{attribute 'no_assign'}
FUNCTION_BLOCK FB_LN_IED_MUnn_LLN0 EXTENDS FB_AcsiCommonLogicalNodeClass
VAR_INPUT
	NamPlt: FB_DO_IED_MUnn_LLN0_NamPlt := (sClass:='LPL', bLinkResult:=THIS^.AddDataToContainer(ipData:=NamPlt));
	Beh: FB_DO_IED_MUnn_LLN0_Beh := (sClass:='ENS', bLinkResult:=THIS^.AddDataToContainer(ipData:=Beh));
	Health: FB_DO_IED_MUnn_LLN0_Health := (sClass:='ENS', bLinkResult:=THIS^.AddDataToContainer(ipData:=Health));
	Mod_: FB_DO_IED_MUnn_LLN0_Mod := (sObjectName:='Mod', sClass:='ENC', bLinkResult:=THIS^.AddDataToContainer(ipData:=Mod_));
	
	PhsMeas1: FB_DS_IED_MUnn_LLN0_PhsMeas1 := (bLinkResult:=THIS^.AddDataSetToContainer(ipDataSet:=PhsMeas1));
	
	MSVCB01: FB_GseMsvCBImplClass := (MsvID:=(sValue:='xxxxMUnn01'), DatSet:=(sValue:='IEDMUnn/LLN0.PhsMeas1'), ConfRev:=(nValue:=1), SmpRate:=(nValue:=80), OptFlds:=(RefreshTime:=TRUE), DstAddress:=(sAddr:='01-0C-CD-04-00-00', nPRIORITY:=4, nVID:=16#000, nAPPID:=16#4000), NoASDU:=(nValue:=1), bLinkResult:=THIS^.AddMulticastSampledValueControlBlockToContainer(ipMulticastSampledValueControlBlock:=MSVCB01));
	MSVCB02: FB_GseMsvCBImplClass := (MsvID:=(sValue:='xxxxMUnn02'), DatSet:=(sValue:='IEDMUnn/LLN0.PhsMeas1'), ConfRev:=(nValue:=1), SmpRate:=(nValue:=256), OptFlds:=(RefreshTime:=TRUE), DstAddress:=(sAddr:='01-0C-CD-04-00-01', nPRIORITY:=4, nVID:=16#000, nAPPID:=16#4001), NoASDU:=(nValue:=8), bLinkResult:=THIS^.AddMulticastSampledValueControlBlockToContainer(ipMulticastSampledValueControlBlock:=MSVCB02));
END_VAR
VAR
END_VAR

END_FUNCTION_BLOCK
